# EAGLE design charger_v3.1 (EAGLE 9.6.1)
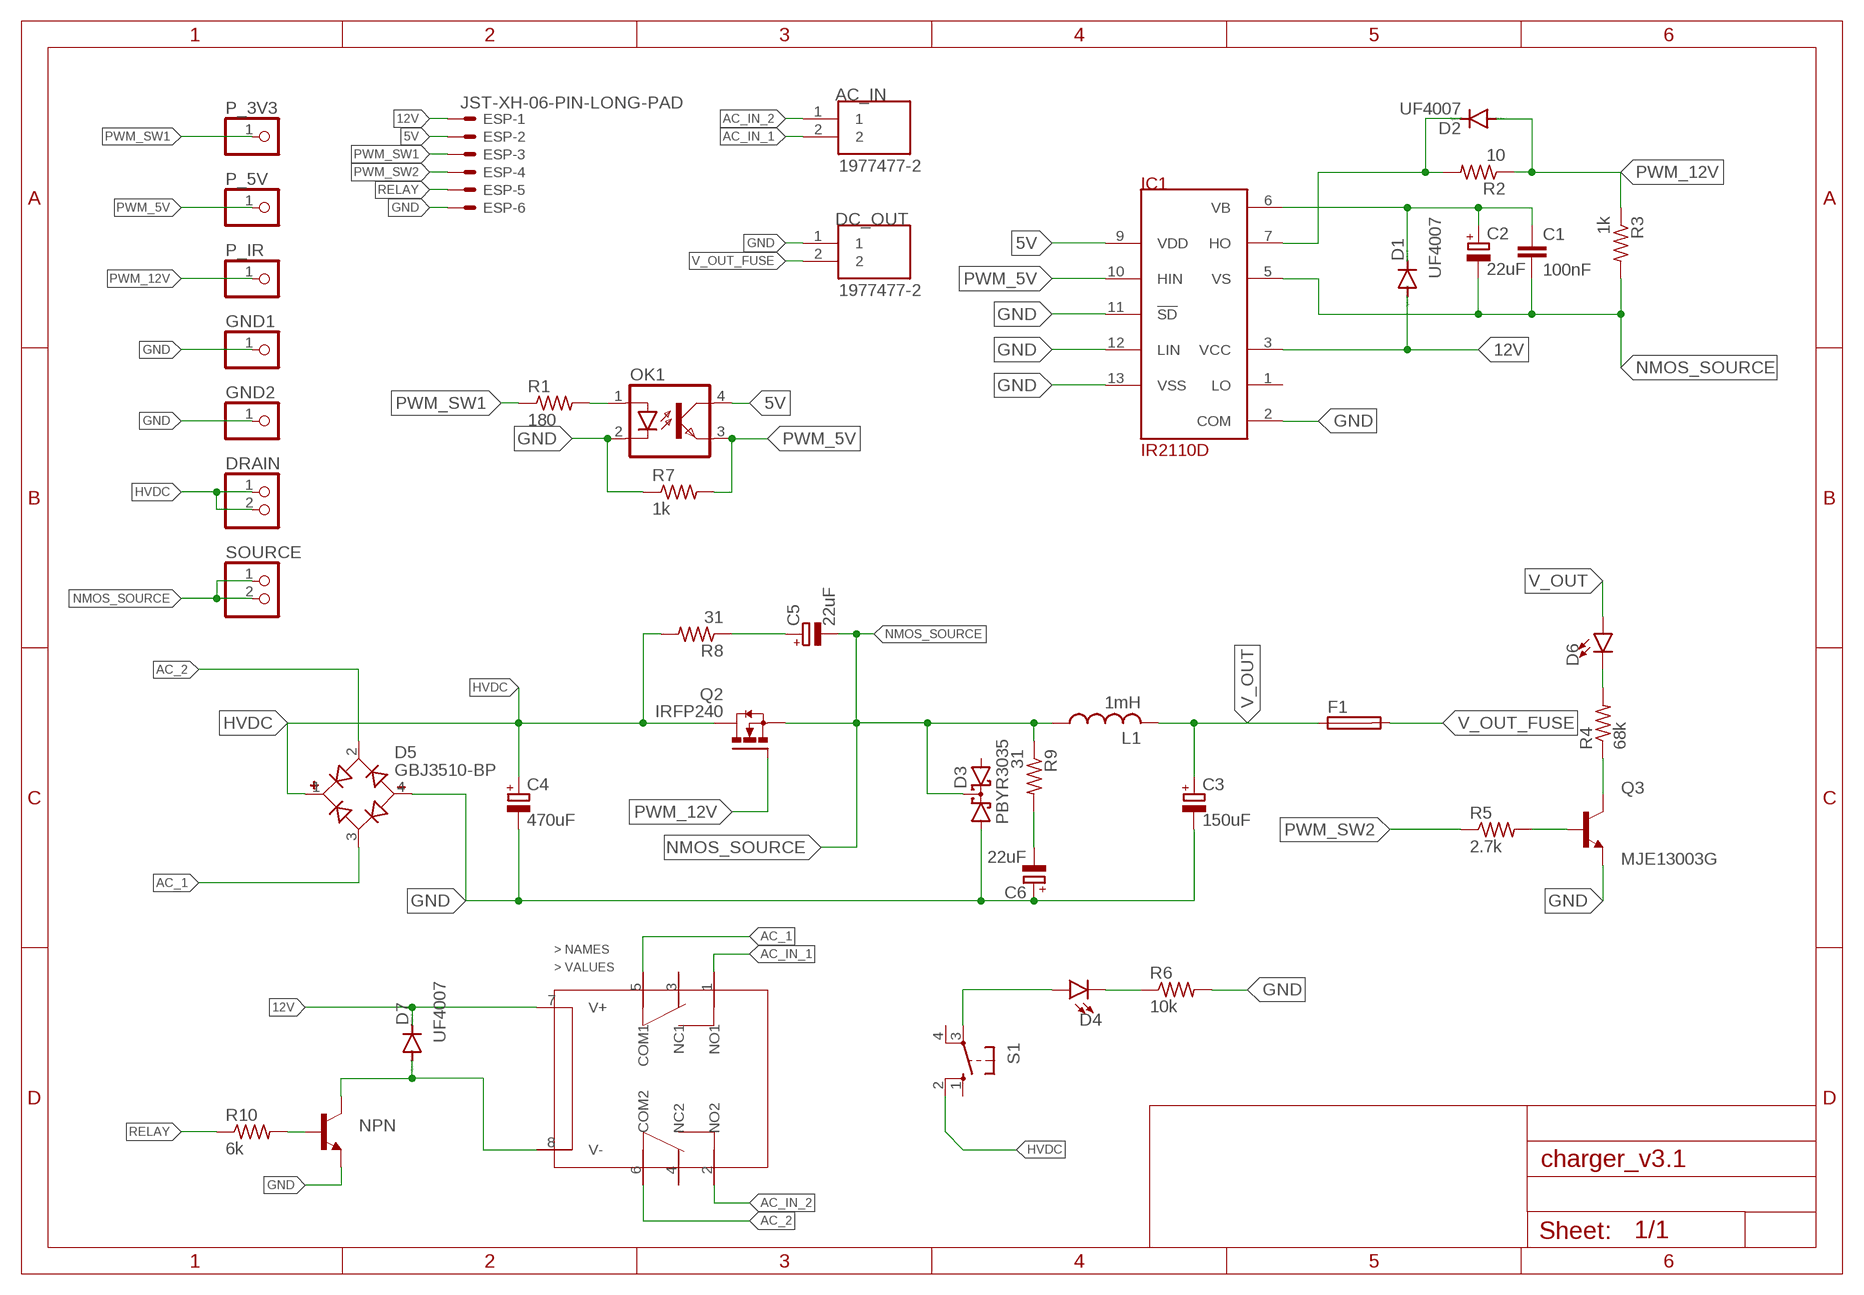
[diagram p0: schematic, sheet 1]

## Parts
AC_IN  1977477-2  [TE_1977477-2]
C1  100nF  C-EU025-025X050  [C025-025X050]
C2  22uF  CPOL-EUE2,5-6E  [E2,5-6E]
C3  150uF  CPOL-EUE7.5-18  [E7,5-18]
C4  470uF  CPOL-EUE10-35  [EB35D]
C5  22uF  CPOL-EUE7.5-18  [E7,5-18]
C6  22uF  CPOL-EUE7.5-18  [E7,5-18]
D1  UF4007  BAS15  [DO34-7]
D2  UF4007  BAS15  [DO34-7]
D3  PBYR3035  [SOT93S]
D4  LED5MM  [LED_5MM]
D5  GBJ3510-BP  [DIOB_GBJ3510-BP]
D6  LED5MM  [LED_5MM]
D7  UF4007  BAS15  [DO34-7]
DC_OUT  1977477-2  [TE_1977477-2]
DRAIN  PINHD-1X2  [1X02]
ESP  JST-XH-06-PIN-LONG-PAD  [JST-XH-06-PACKAGE-LONG-PAD]
F1  FUSEHOLDER  [FUSEHOLDER]
GND1  PINHD-1X1  [1X01]
GND2  PINHD-1X1  [1X01]
IC1  IR2110D  [DIL14]
L1  1mH  L-USTJ7-U1  [TJ7-U1]
NPN  BC547A-NPN-TO92-CBE  [TO92-CBE]
OK1  SFH618A-5  [DIP4]
P_3V3  PINHD-1X1  [1X01]
P_5V  PINHD-1X1  [1X01]
P_IR  PINHD-1X1  [1X01]
Q2  IRFP240  [TO247AC]
Q3  MJE13003G  [TO229P780X300X1364-3]
R1  180  R-US_0204/7  [0204/7]
R2  10  R-US_0204/7  [0204/7]
R3  1k  R-US_0204/7  [0204/7]
R4  68k  R-US_0411/15  [0411/15]
R5  2.7k  R-US_0204/7  [0204/7]
R6  10k  R-US_0204/7  [0204/7]
R7  1k  R-US_0204/7  [0204/7]
R8  31  R-US_0411/15  [0411/15]
R9  31  R-US_0411/15  [0411/15]
R10  6k  R-US_0204/7  [0204/7]
S1  10-XX  [B3F-10XX]
SOURCE  PINHD-1X2  [1X02]
U$1  DPDT-HK19F  [DPDT-HK19F]

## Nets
5V: ESP.2 IC1.9(VDD) OK1.4(COL)
12V: D1.A D7.C ESP.1 IC1.3(VCC) U$1.7(V+)
AC_1: D5.3(AC2) U$1.5(COM1)
AC_2: D5.2(AC1) U$1.6(COM2)
AC_IN_1: AC_IN.2 U$1.1(NO1)
AC_IN_2: AC_IN.1 U$1.2(NO2)
GND: C3.- C4.- C6.+ D3.A1 D5.4(-) DC_OUT.1 ESP.6 GND1.1 GND2.1 IC1.2(COM) IC1.11(!SD) IC1.12(LIN) IC1.13(VSS) NPN.E OK1.2(C) Q3.3(E) R6.2 R7.1
HVDC: C4.+ D5.1(+) DRAIN.1 DRAIN.2 Q2.2(D) R8.2 S1.2(S1)
N$1: D2.C IC1.7(HO) R2.2
N$2: D4.A S1.3(P)
N$3: Q3.2(C) R4.1
N$4: D6.K(C) R4.2
N$5: Q3.1(B) R5.2
N$6: C5.+ R8.1
N$7: C6.- R9.2
N$8: D4.K(C) R6.1
N$9: OK1.1(A) R1.2
N$13: NPN.B R10.2
N$14: D7.A NPN.C U$1.8(V-)
NMOS_SOURCE: C1.2 C2.- C5.- D3.C IC1.5(VS) L1.1 Q2.3(S) R3.2 R9.1 SOURCE.1 SOURCE.2
PWM_5V: IC1.10(HIN) OK1.3(EMIT) P_5V.1 R7.2
PWM_12V [pwm_12]: D2.A P_IR.1 Q2.1(G) R2.1 R3.1
PWM_SW1: ESP.3 P_3V3.1 R1.1
PWM_SW2: ESP.4 R5.1
RELAY: ESP.5 R10.1
V_OUT: C3.+ D6.A F1.1 L1.2
V_OUT_FUSE: DC_OUT.2 F1.2
VB: C1.1 C2.+ D1.C IC1.6(VB)
Unconnected: D3.A2 IC1.1(LO) S1.1(S) S1.4(P1) U$1.3(NC1) U$1.4(NC2)

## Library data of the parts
AC_IN DC_OUT = terminal_block_TA:1977477-2: Check availability; AVAILABILITY: In Stock; COMMENT: 1977477-2; DESCRIPTION: Conn Barrier Strip 2 POS 8.25mm Solder ST Thru-Hole 15A/Contact Carton; MF: TE Connectivity; MP: 1977477-2; PACKAGE: None; PRICE: None; PURCHASE-URL: https://pricing.snapeda.com/search/part/1977477-2/?ref=eda
C1 = rcl:C-EU: CAPACITOR, European symbol; SPICEPREFIX: C
C2-C6 = rcl:CPOL-EU: POLARIZED CAPACITOR, European symbol; SPICEPREFIX: C
D1 D2 D7 = diode:BAS15: DIODE
D3 = diode:PBYR3035: Dual DIODE common cathode
D4 D6 = Sparkfun_LED:LED: LED (Generic)
D5 = GBJ3510-BP:GBJ3510-BP: Diode Rectifier Bridge Single 1KV 35A 4-Pin(4+Tab) Case GBJ Bulk/Tube Check availability; AVAILABILITY: In Stock; DESCRIPTION: Bridge Rectifier Single Phase Standard 1 kV Through Hole GBJ; MF: Micro Commercial; MP: GBJ3510-BP; PACKAGE: SIP-4 Micro Commercial Co; PRICE: None; PURCHASE-URL: https://pricing.snapeda.com/search/part/GBJ3510-BP/?ref=eda
DRAIN SOURCE = pinhead:PINHD-1X2: PIN HEADER
ESP = Rembrandt Electronics - JST XH Connectors v1-0:JST-XH-06-PIN: JST XH Connector 2 Pin Wire to board connector. Pitch: 2,54 mm, (0.100") Number of pins: 6 Created by Rembrandt Electronics www.rembrandtelectronics.com
F1 = TA_library:FUSEHOLDER: FUSE HOLDER; MPN: 0031.7701.11; OC_FARNELL: unknown; OC_NEWARK: 04F1224
GND1 GND2 P_3V3 P_5V P_IR = pinhead:PINHD-1X1: PIN HEADER
IC1 = irs:IR2110
L1 = custom_inductor:L-US: INDUCTOR, American symbol; SPICEPREFIX: L
NPN = transistor:*-NPN-: NPN Transistror BF959 corrected 2008.03.06
OK1 = optocoupler:SFH618?*: Optocoupler, Phototransistor Output, Low Input Current Source: Data sheet; MF: VISHAY/TELEFUNKEN; MPN: SFH618A-5; OC_FARNELL: 1469593; OC_NEWARK: 59K0259
Q2 = IRFP240(TO-247):IRFP240: MOSFET N-CH 200V 20A TO-247AC Check availability; AVAILABILITY: In Stock; DESCRIPTION: N-Channel 200 V 20A (Tc) 150W (Tc) Through Hole TO-247AC; MF: Vishay Siliconix; MP: IRFP240; PACKAGE: TO-247 Vishay Siliconix; PRICE: None
Q3 = MJE13003G:MJE13003G: Bipolar (BJT) Transistor NPN 400V 1.5A 10MHz 1.4W Through Hole TO-225AA Check availability; AVAILABILITY: Not in stock; DESCRIPTION: Bipolar (BJT) Transistor NPN 400 V 1.5 A 10MHz 1.4 W Through Hole TO-126; MF: ON Semiconductor; MP: MJE13003G; PACKAGE: TO-126 ON Semiconductor; PRICE: None
R1-R10 = rcl:R-US_: RESISTOR, American symbol; SPICEPREFIX: R
S1 = switch-omron:10-XX: OMRON SWITCH; MPN: B3F-1000; OC_FARNELL: 176432; OC_NEWARK: 36M3542
U$1 = TA_library:DPDT-HK19F

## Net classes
0 default: width 0.305 mm
1 power: width 6.985 mm, clearance 0.508 mm to class 0
2 pwm_12: width 0.305 mm, clearance 0.508 mm to class 0, clearance 0.508 mm to class 1

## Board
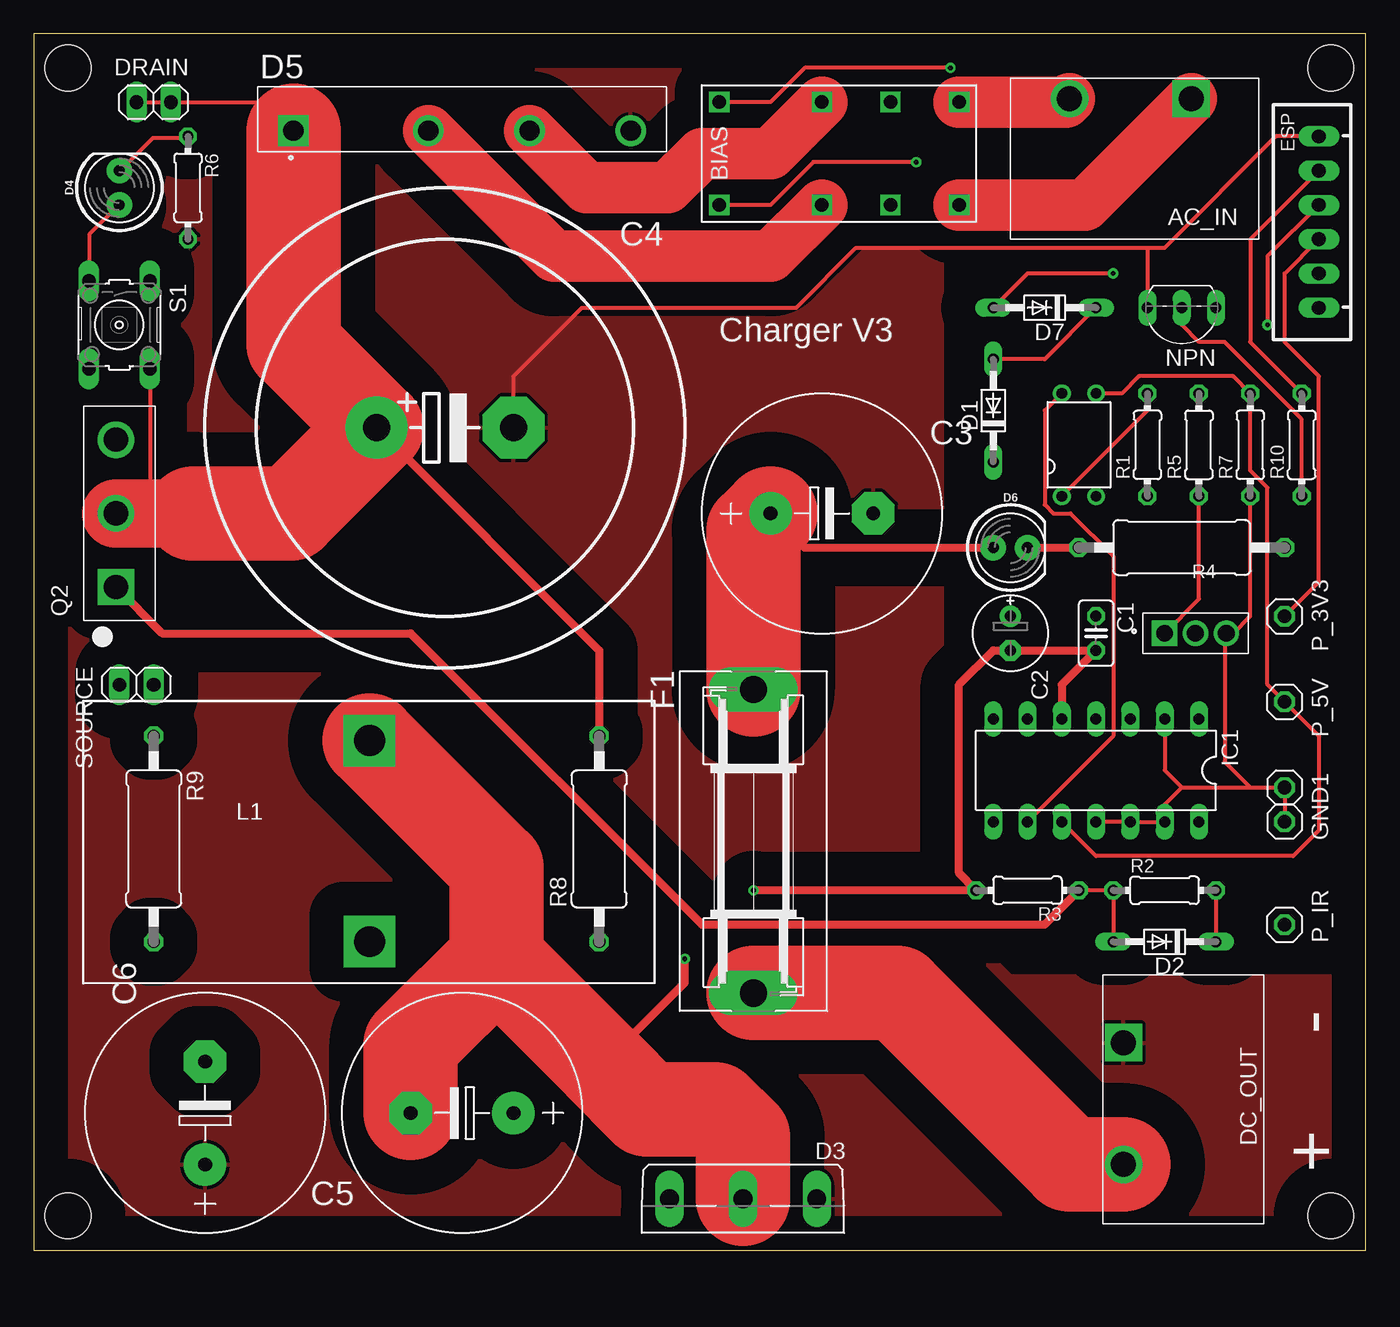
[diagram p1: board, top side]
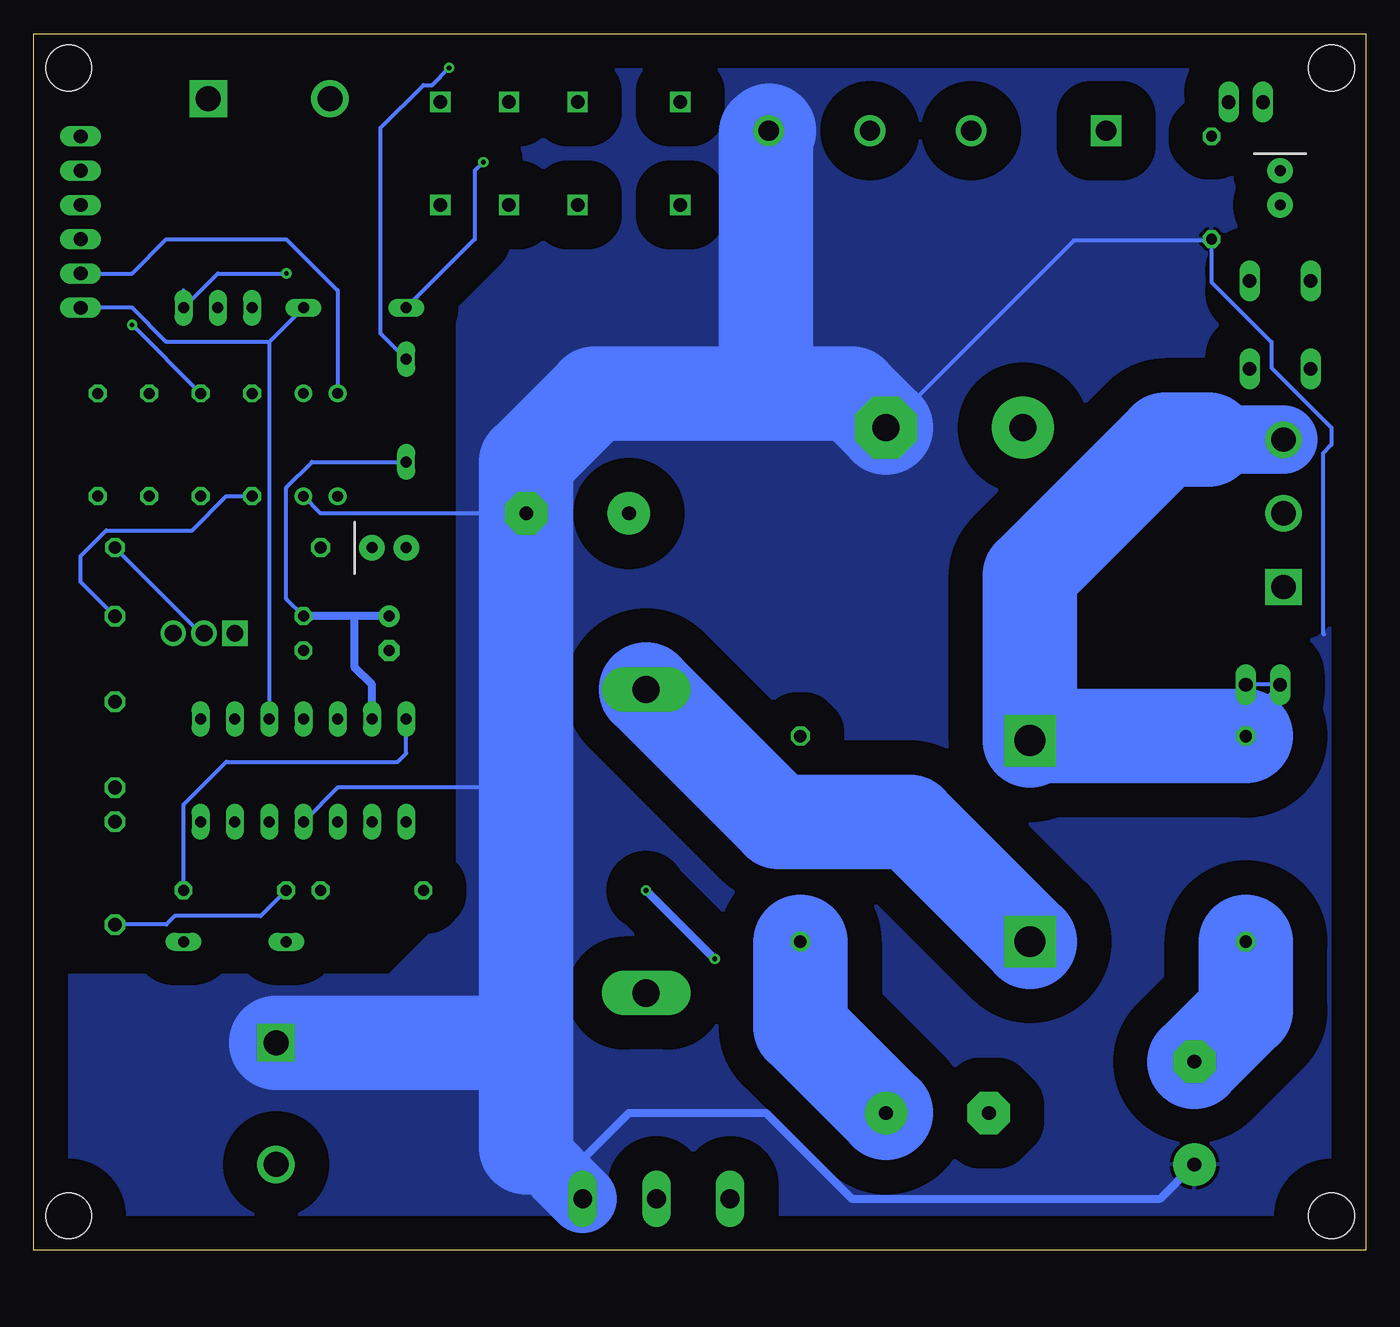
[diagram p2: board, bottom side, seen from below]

Size 98.73 x 90.16 mm. Coordinates in mm from the lower left corner, seen from the top.
Outline: 0,0 98.73,0 98.73,90.16 0,90.16 0,0
Copper layers (1*16): Top 0.035mm / dielectric 1.5mm / Bottom 0.035mm
Design rules "default *": minimum track width 12mil, minimum drill 0.35mm, track to track 12mil, track to pad 12mil, pad to pad 12mil, via to via 12mil, smd to smd 12mil, copper to edge 40mil, drill to drill 6mil, minimum pad ring 10mil, minimum via ring 8mil, stop-mask expansion 4mil, vias tented up to drill 0mil, thermal gap 10mil
Holes 3.4 mm at 2.54,87.63 96.14,87.63 2.54,2.54 96.14,2.54

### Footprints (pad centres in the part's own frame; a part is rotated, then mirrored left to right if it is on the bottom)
TE_1977477-2 = drill 1.85 square: 1 -3.241,-5.334 | drill 1.85: 2 5.781,-5.334
C025-025X050 = drill 0.813 octagon: 1 -1.27,0; 2 1.27,0
E2,5-6E = drill 0.813 pad 1.575: + -1.27,0 | drill 0.813 pad 1.575 octagon: - 1.27,0
E7,5-18 = drill 1.016 pad 3.15: + -3.81,0 | drill 1.016 pad 3.15 octagon: - 3.81,0
EB35D = drill 2.007 pad 4.597: + -5.08,0 | drill 2.007 pad 4.597 octagon: - 5.08,0
DO34-7 = drill 0.813 long: A 3.81,0; C -3.81,0
SOT93S = drill 1.397 long: A1 -5.461,-2.54; A2 5.461,-2.54; C 0,-2.54
LED_5MM = drill 0.813 pad 1.88: A -1.27,0; K 1.27,0
DIOB_GBJ3510-BP = drill 1.51 pad 2.27 square: 1 -12.5,-0.85 | drill 1.51 pad 2.27: 2 -2.5,-0.85; 3 5,-0.85; 4 12.5,-0.85
1X02 = drill 1.016 long: 1 -1.27,0; 2 1.27,0
JST-XH-06-PACKAGE-LONG-PAD = drill 1.016 long: 1 -6.35,0; 2 -3.81,0; 3 -1.27,0; 4 1.27,0; 5 3.81,0; 6 6.35,0
FUSEHOLDER = drill 2.007 pad 3.302 long: 1 -11.252,0; 2 11.252,0
1X01 = drill 1.016 octagon: 1 0,0
DIL14 = drill 0.813 long: 1 -7.62,-3.81; 2 -5.08,-3.81; 3 -2.54,-3.81; 4 0,-3.81; 5 2.54,-3.81; 6 5.08,-3.81; 7 7.62,-3.81; 8 7.62,3.81; 9 5.08,3.81; 10 2.54,3.81; 11 0,3.81; 12 -2.54,3.81; 13 -5.08,3.81; 14 -7.62,3.81
TJ7-U1 = drill 2.286 pad 3.81 square: 1 -6.503,4.826; 2 8.408,4.826
TO92-CBE = drill 0.813 long: B 0,0; C -2.54,0; E 2.54,0
DIP4 = drill 0.8: 1 -1.27,-3.81; 2 1.27,-3.81; 3 1.27,3.81; 4 -1.27,3.81
TO247AC = drill 1.79 pad 2.69 square: 1 -5.46,0.255 | drill 1.79 pad 2.69: 2 0,0.255; 3 5.46,0.255
TO229P780X300X1364-3 = drill 1.25 square: 1 0,0 | drill 1.25: 2 2.29,0; 3 4.58,0
0204/7 = drill 0.813 octagon: 1 -3.81,0; 2 3.81,0
0411/15 = drill 0.914 octagon: 1 -7.62,0; 2 7.62,0
B3F-10XX = drill 1.016 long: 1 -3.251,2.261; 2 3.251,2.261; 3 -3.251,-2.261; 4 3.251,-2.261
DPDT-HK19F = drill 1 square: 1 8.89,3.81; 2 8.89,-3.81; 3 3.81,3.81; 4 3.81,-3.81; 5 -1.27,3.81; 6 -1.27,-3.81; 7 -8.89,3.81; 8 -8.89,-3.81

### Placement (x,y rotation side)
AC_IN  82.55,80.01 180 top
C1  78.74,45.72 270 top
C2  72.39,45.72 270 top
C3  58.42,54.61 0 top
C4  30.48,60.96 0 top
C5  31.75,10.16 180 top
C6  12.7,10.16 90 top
D1  71.12,62.23 90 top
D2  83.82,22.86 180 top
D3  52.58,1.27 180 top
D4  6.35,78.74 90 top
D5  31.75,83.82 0 top
D6  72.39,52.07 0 top
D7  74.93,69.85 180 top
DC_OUT  86.11,12.13 270 top
DRAIN  8.89,85.09 180 top
ESP  95.25,76.2 90 top
F1  53.34,30.3 270 top
GND1  92.71,31.75 0 top
GND2  92.71,34.29 0 top
IC1  78.74,35.56 180 top
L1  20.07,31.27 270 top
NPN  85.09,69.85 180 top
OK1  77.47,59.69 0 top
P_3V3  92.71,46.99 90 top
P_5V  92.71,40.64 90 top
P_IR  92.71,24.13 90 top
Q2  6.35,54.61 90 top
Q3  83.82,45.72 0 top
R1  82.55,59.69 90 top
R2  83.82,26.67 0 top
R3  73.66,26.67 180 top
R4  85.09,52.07 180 top
R5  86.36,59.69 270 top
R6  11.43,78.74 270 top
R7  90.17,59.69 90 top
R8  41.91,30.48 90 top
R9  8.89,30.48 270 top
R10  93.98,59.69 270 top
S1  6.35,68.58 270 top
SOURCE  7.62,41.91 180 top
U$1  59.69,81.28 0 top

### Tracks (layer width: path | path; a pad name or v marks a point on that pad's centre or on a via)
5V
  Top 0.305: IC1.9 80.01,38.1 80.01,51.43 76.83,54.61 75.56,54.61 74.93,55.24 74.93,62.23 OK1.4
  Bottom 0.305: OK1.4 76.2,71.12 80.01,74.93 88.9,74.93 91.44,72.39 ESP.2
12V  (via drill 0.35)
  Top 0.305: D1.A 74.93,66.04 D7.C | U$1.7 54.61,85.09 57.15,87.63 v67.94,87.63
  Bottom 0.305: 81.28,67.31 IC1.3 | D7.C 81.28,67.31 | v67.94,87.63 69.22,86.36 69.85,86.36 73.03,83.19 73.03,67.95 D1.A | ESP.1 91.44,69.85 88.9,67.31 81.28,67.31
AC_1
  Top 3.81: D5.3 40.98,78.74 46.99,78.74 49.53,81.28 54.61,81.28 U$1.5
AC_2
  Top 3.81: U$1.6 54.61,73.66 38.56,73.66 D5.2
AC_IN_1
  Top 3.81: U$1.1 76.52,85.09 AC_IN.2
AC_IN_2
  Top 3.81: U$1.2 77.92,77.47 AC_IN.1
GND
  Top 0.305: 35.66,60.96 C4.- | ESP.6 92.08,82.55 83.82,74.3 82.55,74.3 | R7.1 90.17,46.99 88.9,45.72 Q3.3 88.27,45.72 88.27,36.2 90.17,34.29 | GND1.1 GND2.1 90.17,34.29 | IC1.11 IC1.12 IC1.13 83.82,33.02 85.09,34.29 | 82.55,74.3 60.96,74.3 56.52,69.85 40.64,69.85 35.56,64.77 C4.- | 82.55,74.3 NPN.E | 35.56,59.05 C4.- | IC1.2 83.82,35.56 85.09,34.29 | 85.09,34.29 90.17,34.29
  Bottom 0.305: C4.- 35.51,60.96 21.64,74.83 11.43,74.83 R6.2 11.43,71.76 6.99,67.31 6.99,65.41 2.54,60.96 2.54,59.69 3.17,59.05 3.17,45.72 3.1,45.65 | 44.2,82.91 D5.4 46.85,80.37 | D3.A1 58.04,6.25 | 12.8,6.25 C6.+ | OK1.2 77.47,54.61 C3.- | 62.23,31.75 64.77,34.29 76.2,34.29 IC1.11 | 62.36,15.37 62.23,15.24
  Bottom 0.61: D3.A1 58.04,6.73 54.61,10.16 44.45,10.16 38.1,3.81 15.24,3.81 12.8,6.25
  Bottom 5.08: D3.A1 61.85,7.62 62.23,7.62
  Bottom 6.985: C4.- 38.1,63.5 44.45,63.5 | D5.4 44.45,82.77 44.45,63.5 | 44.45,63.5 57.15,63.5 62.23,58.42 C3.- 62.23,31.75 62.23,15.24 62.23,7.62 | DC_OUT.1 62.36,15.37
  pour Top (isolate 2.54): -10.16,95.25 69.85,95.25 69.85,76.2 67.31,73.66 67.31,25.4 72.39,20.32 97.79,20.32 99.06,19.05 99.06,-7.62 -10.16,-7.62
  pour Bottom (isolate 2.54): -12.7,97.79 69.85,97.79 69.85,76.2 67.31,73.66 67.31,25.4 72.39,20.32 97.79,20.32 99.06,19.05 99.06,-7.62 -12.7,-7.62
HVDC
  Top 0.305: 8.69,54.61 8.69,56.99 | 8.69,56.99 8.69,65.23 S1.2 | 8.69,56.99 8.73,56.99 8.73,54.61 | D5.1 17.13,85.09 DRAIN.1 DRAIN.2
  Top 0.61: R8.2 41.91,44.45 C4.+
  Top 5.08: Q2.2 8.73,54.61 11.81,54.61
  Top 6.985: D5.1 19.25,67.11 C4.+ 19.05,54.61 11.81,54.61
N$1
  Top 0.305: R2.2 D2.C
  Bottom 0.305: IC1.7 71.12,36.83 71.75,36.2 84.45,36.2 87.63,33.02 R2.2
N$2
  Top 0.305: S1.3 4.12,71.93 4.12,75.29 6.25,77.42 D4.A
N$3
  Bottom 0.305: R4.1 86.36,45.72 Q3.2
N$4
  Top 0.61: D6.K R4.2
N$5
  Top 0.305: R5.2 86.36,48.26 Q3.1
N$6
  Bottom 6.985: R8.1 41.91,16.51 C5.+
N$7
  Bottom 6.985: C6.- 8.89,17.78 R9.2
N$8
  Top 0.305: R6.1 11.43,82.45 8.84,82.45 6.4,80.01 D4.K
N$9
  Top 0.305: R1.2 82.55,62.23 OK1.1
N$13
  Top 0.305: R10.2 93.98,61.59 88.27,67.31 86.36,67.31 85.09,68.58 NPN.B
N$14  (via drill 0.35)
  Top 0.305: v80.01,72.39 73.66,72.39 D7.A | U$1.8 54.61,77.47 57.78,80.65 v65.41,80.65
  Bottom 0.305: v65.41,80.65 66.04,80.01 66.04,74.93 D7.A | 87.63,71.12 NPN.C 85.09,72.39 v80.01,72.39
NMOS_SOURCE  (via drill 0.35)
  Top 0.61: IC1.5 76.2,41.91 C1.2 C2.- 71.12,44.45 68.58,41.91 68.58,27.94 R3.2 v53.34,26.67 | 42.15,13.73 48.26,19.84 v48.26,21.59
  Top 6.985: L1.1 34.29,28.37 34.29,21.59 | 34.29,21.59 42.15,13.73 45.43,10.45 50.51,10.45 52.58,8.38 D3.C | C5.- 27.94,15.24 34.29,21.59
  Bottom 0.305: R9.1 8.89,39.37 SOURCE.2 SOURCE.1
  Bottom 0.61: v48.26,21.59 v53.34,26.67
  Bottom 5.08: Q2.3 11.68,60.07
  Bottom 6.985: 11.68,60.07 14.86,60.07 24.89,50.04 L1.1 24.56,38.1 R9.1
PWM_5V
  Top 0.305: OK1.3 80.64,63.5 81.92,64.77 88.9,64.77 R7.2 90.17,57.78 91.44,56.52 91.44,41.91 P_5V.1 95.25,38.1 95.25,31.12 93.34,29.21 78.74,29.21 IC1.10
PWM_12V
  Top 0.305: R3.1 R2.1 D2.A
  Top 0.61: Q2.1 9.53,45.72 27.94,45.72 49.53,24.13 74.93,24.13 R3.1
  Bottom 0.305: P_IR.1 88.9,24.13 88.27,24.77 81.92,24.77 R2.1
PWM_SW1
  Top 0.305: ESP.3 92.71,72.39 92.71,67.31 95.25,64.77 95.25,49.53 P_3V3.1
  Bottom 0.305: R1.1 84.45,55.88 87,53.34 93.34,53.34 95.25,51.43 95.25,49.53 P_3V3.1
PWM_SW2  (via drill 0.35)
  Top 0.305: v91.44,68.58 91.44,73.66 ESP.4
  Bottom 0.305: v91.44,68.58 R5.1
RELAY
  Top 0.305: R10.1 90.17,67.31 90.17,74.93 ESP.5
V_OUT
  Top 0.61: C3.+ 57.15,52.07 D6.A
  Top 6.985: C3.+ 53.34,53.34 F1.1
  Bottom 6.985: L1.2 33.78,31.75 43.54,31.75 F1.1
V_OUT_FUSE
  Top 6.985: F1.2 64.01,19.05 76.71,6.35 DC_OUT.2
VB
  Bottom 0.305: D1.C 78.11,58.42 80.01,56.52 80.01,48.26 C1.1
  Bottom 0.61: IC1.6 73.66,41.91 74.93,43.18 74.93,46.99 | 74.93,46.99 C1.1 | C2.+ 74.93,46.99

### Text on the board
tPlace: - | +
tNames: Charger V3

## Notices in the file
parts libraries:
Sparkfun_LED: Licensing: Creative Commons ShareAlike 4.0 International - https://creativecommons.org/licenses/by-sa/4.0
